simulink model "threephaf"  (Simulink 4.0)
settings: Solver=ode23  StartTime=-eps  StopTime=0.1  FixedStep=0.000001  MaxStep=2e-5  RelTol=1e-3
undefined symbols (not defined in the file or in its folder): Cdc, di, Element, L, R, sfunxy, Symmetrized, Tf, Ts, Udc, Upp, Warning, Yes
libraries: simulink3 x7
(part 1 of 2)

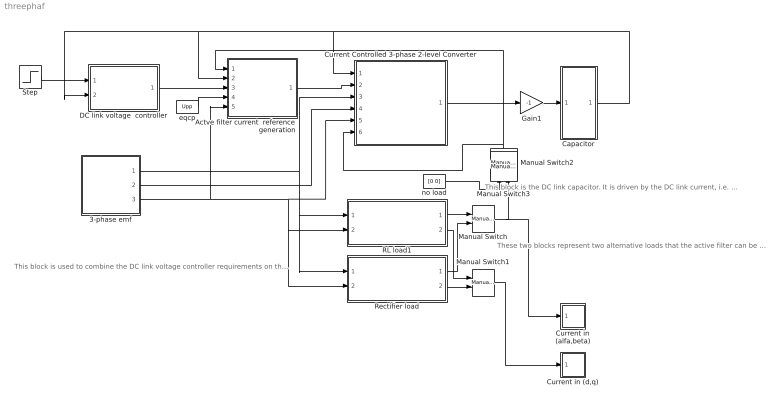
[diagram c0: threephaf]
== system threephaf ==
  note: These two blocks represent two alternative loads that the active filter can be used with.
  note: This block is the DC link capacitor. It is driven by the DC link current, i.e. the DC link voltage is the integral of the DC link current divided by the capacitance.
  note: This block is used to combine the DC link voltage controller requirements on the filter current with the components of the load current that can be filtered out.
  3-phase emf : Subsystem  SimViewingDevice=off  mask{Upp=Upp, freq=50, Tc=0.1e-3}
      mask prompts: Upp "U_phase_to_phase [RMS]"; freq "Frequency"; Tc "Sampling time"
  Actve filter current  reference generation : Subsystem  SimViewingDevice=off
  Capacitor : Subsystem  SimViewingDevice=off
  Current Controlled 3-phase 2-level Converter : Subsystem  SimViewingDevice=off
  Current in (alfa,beta) : Subsystem  LoadFcn=sfunxy([],[],[],'LoadBlock')  StartFcn=sfunxy([],[],[],'Start')  StopFcn=sfunxy([],[],[],'Stop')  SimViewingDevice=off  mask(XY scope.){xmin=-20, xmax=20, ymin=-20, ymax=20, st=-1}
      mask prompts: xmin "x-min:"; xmax "x-max:"; ymin "y-min:"; ymax "y-max:"; st "Sample time:"
      mask help: XY scope using MATLAB graph window. First input is used as time base. Enter plotting ranges.
  Current in (d,q) : Subsystem  LoadFcn=sfunxy([],[],[],'LoadBlock')  StartFcn=sfunxy([],[],[],'Start')  StopFcn=sfunxy([],[],[],'Stop')  SimViewingDevice=off  mask(XY scope.){xmin=-20, xmax=20, ymin=-20, ymax=20, st=-1}
      mask prompts: xmin "x-min:"; xmax "x-max:"; ymin "y-min:"; ymax "y-max:"; st "Sample time:"
      mask help: XY scope using MATLAB graph window. First input is used as time base. Enter plotting ranges.
  DC link voltage  controller : Subsystem  SimViewingDevice=off  mask{Kp=Cdc/3/Tf, Ti=9*Tf, Ttc=Ts, Limitoutput=Yes, Out_max=20, Out_min=-20}
      mask prompts: Kp "Gain"; Ti "Integral time constant"; Ttc "Controller Sampling Time"; Limitoutput "Limit the output"; Out_max "Max Controller Output (if limited)     INCLUDES Anti Windup !!"; Out_min "Min Controller Output (if limited)     INCLUDES Anti Windup !!"
  Gain1 : Gain  Gain=-1  Multiplication=Element-wise(K.*u)  SaturateOnIntegerOverflow=on
  Manual Switch : simulink3/Nonlinear/Manual Switch  sw=0  action=0
  Manual Switch1 : simulink3/Nonlinear/Manual Switch  sw=0  action=0
  Manual Switch2 : simulink3/Nonlinear/Manual Switch  Orientation=up  sw=0  action=0
  Manual Switch3 : simulink3/Nonlinear/Manual Switch  Orientation=up  sw=0  action=0
  RL load1 : Subsystem  SimViewingDevice=off  mask{Ra=5, Rb=5, Rc=5, La=0.005, Lb=0.005, Lc=0.005, Imax=1}
      mask prompts: Ra "Ra [Ohm]"; Rb "Rb [Ohm]"; Rc "Rc [Ohm]"; La "La [H]"; Lb "Lb [H]"; Lc "Lc [H]"; Imax "Current when saturation starts"
  Rectifier load : Subsystem  SimViewingDevice=off
  Step : Step  Time=0.005  Before=250  After=260  SampleTime=0
  eqcp : Constant  Value=Upp
  no load : Constant  Value=[0 0]
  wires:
  Gain1/1 -> Capacitor/1(iC)
  Current Controlled 3-phase 2-level Converter/1(idc) -> Gain1/1
  DC link voltage  controller/1(Out) -> Actve filter current  reference generation/3(idc*)
  eqcp/1 -> Actve filter current  reference generation/4(eqcp)
  Step/1 -> DC link voltage  controller/1(Ref)
  Capacitor/1(Udc) -> Actve filter current  reference generation/2(Udc), DC link voltage  controller/2(Act), Current Controlled 3-phase 2-level Converter/1(Udc)
  RL load1/1(i_load_ab) -> Manual Switch/1
  Rectifier load/1(i_load_ab) -> Manual Switch/2
  Rectifier load/2(i_load_dq) -> Manual Switch1/2
  RL load1/2(i_load_dq) -> Manual Switch1/1
  Actve filter current  reference generation/1(idq*) -> Current Controlled 3-phase 2-level Converter/2(idq*)
  3-phase emf/1(e_line) -> Current Controlled 3-phase 2-level Converter/3(e_line), Rectifier load/1(u_line), RL load1/1(u_line)
  3-phase emf/2(Psi_line) -> Current Controlled 3-phase 2-level Converter/4(Psi_line)
  3-phase emf/3(Theta_line) -> Actve filter current  reference generation/5(Theta), Current Controlled 3-phase 2-level Converter/5(Theta_line), Rectifier load/2(Theta), RL load1/2(Theta)
  Manual Switch/1 -> Manual Switch2/2, Current in (alfa,beta)/1(xy)
  no load/1 -> Manual Switch2/1
  Manual Switch2/1 -> Actve filter current  reference generation/1(i_load), Current Controlled 3-phase 2-level Converter/6(Load current in a/b)
  Manual Switch1/1 -> Current in (d,q)/1(xy)

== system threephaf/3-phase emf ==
  note: Power invariant emf vector on alpha/beta frame
  Cos Fcn : Fcn  Expr=cos(2*pi*(u(2))*u(1))
  Digital Clock : DigitalClock  SampleTime=Tc
  Mux : Mux  Inputs=2
  Mux1 : Mux  Inputs=2
  Product : Product  Inputs=2  Multiplication=Element-wise(.*)  SaturateOnIntegerOverflow=on
  Sine Fcn : Fcn  Expr=sin(2*pi*(u(2))*u(1)-pi)
  frequency : Constant  Value=freq
  integrator : Subsystem  SimViewingDevice=off
  line voltage : Constant  Value=Upp
  rec_to_pol : Subsystem  SimViewingDevice=off
  e_line : Outport  Port=1  InitialOutput=0
  Psi_line : Outport  Port=2  InitialOutput=0
  Theta_line : Outport  Port=3  InitialOutput=0
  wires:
  Product/1 -> e_line/1, integrator/1(In1)
  Mux1/1 -> Product/1
  Cos Fcn/1 -> Mux1/2
  Sine Fcn/1 -> Mux1/1
  Mux/1 -> Cos Fcn/1, Sine Fcn/1
  Digital Clock/1 -> Mux/1
  frequency/1 -> Mux/2
  line voltage/1 -> Product/2
  integrator/1(Out1) -> Psi_line/1, rec_to_pol/1(rect)
  rec_to_pol/2(angle) -> Theta_line/1

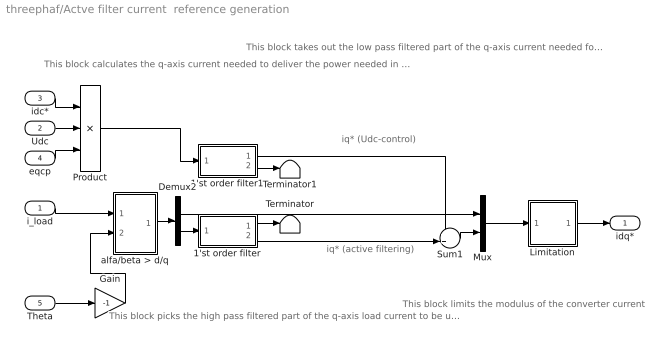
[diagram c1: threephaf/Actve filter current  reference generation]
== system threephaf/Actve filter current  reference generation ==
  note: iq* (Udc-control)
  note: iq* (active filtering)
  note: This block calculates the q-axis current needed to deliver the power needed in the dc-link for correcting the DC link voltage error, as ordered by the DC link voltage controller
  note: This block takes out the low pass filtered part of the q-axis current needed for DC link voltage control
  note: This block picks the high pass filtered part of the q-axis load current to be used as reference for the q-axis together with the low pass filtered part of the DC link voltage controller output.
  note: This block limits the modulus of the converter current
  i_load : Inport  Port=1  PortDimensions=-1  SampleTime=-1  DataType=auto
  Udc : Inport  Port=2  PortDimensions=-1  SampleTime=-1  DataType=auto
  idc* : Inport  Port=3  PortDimensions=-1  SampleTime=-1  DataType=auto
  eqcp : Inport  Port=4  PortDimensions=-1  SampleTime=-1  DataType=auto
  Theta : Inport  Port=5  PortDimensions=-1  SampleTime=-1  DataType=auto
  1'st order filter : Subsystem  SimViewingDevice=off
  1'st order filter1 : Subsystem  SimViewingDevice=off
  Demux2 : Demux  Outputs=2  BusSelectionMode=off
  Gain : Gain  Gain=-1  Multiplication=Element-wise(K.*u)  SaturateOnIntegerOverflow=on
  Limitation : Subsystem  SimViewingDevice=off
  Mux : Mux  Inputs=2
  Product : Product  Inputs=**/  Multiplication=Element-wise(.*)  SaturateOnIntegerOverflow=on
  Sum1 : Sum  Inputs=++|  SaturateOnIntegerOverflow=on
  Terminator : Terminator
  Terminator1 : Terminator
  alfa/beta > d/q : Subsystem  SimViewingDevice=off
  idq* : Outport  Port=1
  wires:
  i_load/1 -> alfa/beta > d/q/1(vect)
  Gain/1 -> alfa/beta > d/q/2(angle)
  Theta/1 -> Gain/1
  Demux2/1 -> Mux/1
  Demux2/2 -> 1'st order filter/1(In)
  1'st order filter/1(OutLP) -> Terminator/1
  alfa/beta > d/q/1(Out) -> Demux2/1
  1'st order filter/2(OutHP) -> Sum1/2
  Sum1/1 -> Mux/2
  Limitation/1(i*lim) -> idq*/1
  1'st order filter1/1(OutLP) -> Sum1/1
  eqcp/1 -> Product/3
  Udc/1 -> Product/2
  Product/1 -> 1'st order filter1/1(In)
  idc*/1 -> Product/1
  1'st order filter1/2(OutHP) -> Terminator1/1
  Mux/1 -> Limitation/1(i*)

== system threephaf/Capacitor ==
  iC : Inport  Port=1  PortDimensions=-1  SampleTime=-1  DataType=auto
  Gain : Gain  Gain=1/Cdc  Multiplication=Element-wise(K.*u)  SaturateOnIntegerOverflow=on
  Integrator : Integrator  ExternalReset=none  InitialConditionSource=internal  InitialCondition=Udc  LimitOutput=off  UpperSaturationLimit=inf  LowerSaturationLimit=-inf  ShowSaturationPort=off  ShowStatePort=off  AbsoluteTolerance=auto
  Udc : Outport  Port=1
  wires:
  Gain/1 -> Integrator/1
  iC/1 -> Gain/1
  Integrator/1 -> Udc/1

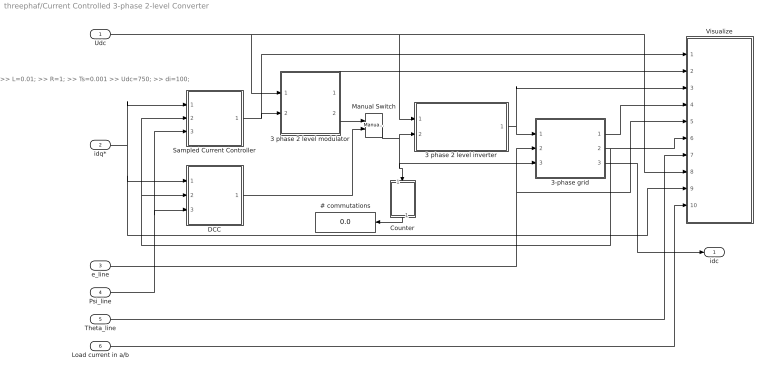
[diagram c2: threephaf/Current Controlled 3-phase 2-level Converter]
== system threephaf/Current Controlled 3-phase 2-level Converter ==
  note: >> L=0.01; >> R=1; >> Ts=0.001 >> Udc=750; >> di=100;
  Udc : Inport  Port=1  PortDimensions=-1  SampleTime=-1  DataType=auto
  idq* : Inport  Port=2  PortDimensions=-1  SampleTime=-1  DataType=auto
  e_line : Inport  Port=3  PortDimensions=-1  SampleTime=-1  DataType=auto
  Psi_line : Inport  Port=4  PortDimensions=-1  SampleTime=-1  DataType=auto
  Theta_line : Inport  Port=5  PortDimensions=-1  SampleTime=-1  DataType=auto
  Load current in a/b : Inport  Port=6  PortDimensions=-1  SampleTime=-1  DataType=auto
  # commutations : Display
  3 phase 2 level inverter : Subsystem  SimViewingDevice=off
  3 phase 2 level modulator : Subsystem  SimViewingDevice=off  mask{type=Symmetrized, Random=Fixed frequency, Ts=Ts}
      mask prompts: type "Sinus, Symmetrized or Minimum switch modulation"; Random "Fixed or random modulation?"; Ts "Sampling interval"
      mask help: Carrier Wave modulator that uses either fixed frequency modulation or random modulation. The fixed frequency modulation uses 1/(2Ts) as modulation frequency. The random modulation selects the modulatio frequency by random every sampling instant. The selection uses either 1/Ts, 1/(2Ts) or 1/(3Ts) as carrier wave frequency.
  3-phase grid : Subsystem  SimViewingDevice=off  mask{L=L, R=R}
      mask prompts: L "Inductance [H]"; R "Resistance [ohm]"
  Counter : Subsystem  Orientation=down  SimViewingDevice=off
  DCC : Subsystem  SimViewingDevice=off
  Manual Switch : simulink3/Nonlinear/Manual Switch  sw=1  action=0
  Sampled Current Controller : Subsystem  SimViewingDevice=off  mask{R=R, L=L, Kp=(L/Ts+R/2), Ti=L/R+Ts/2, Ts=Ts, Umax=Udc, Umin=-Udc, SlowFast=Fast computer}
      mask prompts: R "Load resistance"; L "Load inductance"; Kp "Controller gain"; Ti "Integral Time Constant"; Ts "Sampling time [s]"; Umax "Max output signal"; Umin "Min output signal"; SlowFast "Controller type"
  Visualize : Subsystem  SimViewingDevice=off
  idc : Outport  Port=1
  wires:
  3 phase 2 level inverter/1(va,b,c) -> 3-phase grid/1(va,b,c), Visualize/3(v)
  Sampled Current Controller/1(u*) -> 3 phase 2 level modulator/2(uabc*), Visualize/1(u*)
  Udc/1 -> 3 phase 2 level modulator/1(Udc), 3 phase 2 level inverter/1(Udc), Visualize/8(Udc)
  Counter/1(#) -> # commutations/1
  3 phase 2 level modulator/2(sa,b,c) -> Manual Switch/1
  Manual Switch/1 -> 3 phase 2 level inverter/2(sa,b,c), Counter/1(sa,b,c), 3-phase grid/3(s)
  DCC/1(sa,b,c) -> Manual Switch/2
  3 phase 2 level modulator/1(mod) -> Visualize/2(mod)
  e_line/1 -> 3-phase grid/2(e_line), Visualize/5(e)
  3-phase grid/1(u_ab) -> Visualize/4("u ")
  3-phase grid/2(i_ab) -> Visualize/6(i), DCC/2(Act_ab), Sampled Current Controller/2(Act_ab)
  Theta_line/1 -> Visualize/7(theta)
  Psi_line/1 -> DCC/3(psi), Sampled Current Controller/3(psi)
  idq*/1 -> Sampled Current Controller/1(Ref_dq), DCC/1(Ref_dq), Visualize/9(i*dq)
  3-phase grid/3(i_dc) -> idc/1
  Load current in a/b/1 -> Visualize/10(Load current in a/b)

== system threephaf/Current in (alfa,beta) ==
  xy : Inport  Port=1  PortDimensions=-1  SampleTime=-1  DataType=auto
  sfunxy : S-Function  FunctionName=sfunxy  Parameters=[xmin xmax ymin ymax], st  PortCounts=[]  SFunctionModules=''
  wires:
  xy/1 -> sfunxy/1

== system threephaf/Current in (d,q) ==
  xy : Inport  Port=1  PortDimensions=-1  SampleTime=-1  DataType=auto
  sfunxy : S-Function  FunctionName=sfunxy  Parameters=[xmin xmax ymin ymax], st  PortCounts=[]  SFunctionModules=''
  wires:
  xy/1 -> sfunxy/1

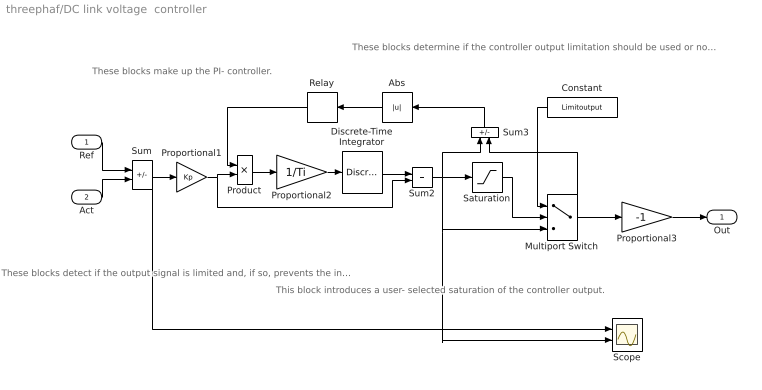
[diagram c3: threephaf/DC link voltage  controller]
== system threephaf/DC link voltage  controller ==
  note: These blocks make up the PI- controller.
  note: These blocks detect if the output signal is limited and, if so, prevents the integrator from integrating.
  note: This block introduces a user- selected saturation of the controller output.
  note: These blocks determine if the controller output limitation should be used or not.
  Ref : Inport  Port=1  PortDimensions=-1  SampleTime=-1  DataType=auto
  Act : Inport  Port=2  PortDimensions=-1  SampleTime=-1  DataType=auto
  Abs : Abs  Orientation=left  SaturateOnIntegerOverflow=on
  Constant : Constant  Orientation=left  Value=Limitoutput
  Discrete-Time Integrator : DiscreteIntegrator  IntegratorMethod=Forward Euler  ExternalReset=none  InitialConditionSource=internal  InitialCondition=0  LimitOutput=off  UpperSaturationLimit=inf  LowerSaturationLimit=-inf  ShowSaturationPort=off  ShowStatePort=off  SampleTime=Ttc
  Multiport Switch : MultiPortSwitch  Inputs=2
  Product : Product  Inputs=2  Multiplication=Element-wise(.*)  SaturateOnIntegerOverflow=on
  Proportional1 : Gain  Gain=Kp  Multiplication=Element-wise(K.*u)  SaturateOnIntegerOverflow=on
  Proportional2 : Gain  Gain=1/Ti  Multiplication=Element-wise(K.*u)  SaturateOnIntegerOverflow=on
  Proportional3 : Gain  Gain=-1  Multiplication=Element-wise(K.*u)  SaturateOnIntegerOverflow=on
  Relay : Relay  Orientation=left  OnSwitchValue=eps  OffSwitchValue=eps  OnOutputValue=0  OffOutputValue=1
  Saturation : Saturate  UpperLimit=Out_max  LowerLimit=Out_min  LinearizeAsGain=on
  Scope : Scope  NumInputPorts=2
  Sum : Sum  Inputs=+-  SaturateOnIntegerOverflow=on
  Sum2 : Sum  Inputs=++  SaturateOnIntegerOverflow=on
  Sum3 : Sum  Orientation=up  Inputs=+-  SaturateOnIntegerOverflow=on
  Out : Outport  Port=1
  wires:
  Sum/1 -> Proportional1/1, Scope/1
  Discrete-Time Integrator/1 -> Sum2/1
  Proportional1/1 -> Product/2, Sum2/2
  Proportional2/1 -> Discrete-Time Integrator/1
  Sum2/1 -> Saturation/1, Sum3/1, Multiport Switch/3, Scope/2
  Product/1 -> Proportional2/1
  Sum3/1 -> Abs/1
  Abs/1 -> Relay/1
  Relay/1 -> Product/1
  Ref/1 -> Sum/1
  Act/1 -> Sum/2
  Saturation/1 -> Multiport Switch/2
  Constant/1 -> Multiport Switch/1
  Multiport Switch/1 -> Sum3/2, Proportional3/1
  Proportional3/1 -> Out/1

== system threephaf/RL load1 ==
  u_line : Inport  Port=1  PortDimensions=-1  SampleTime=-1  DataType=auto
  Theta : Inport  Port=2  PortDimensions=-1  SampleTime=-1  DataType=auto
  Gain1 : Gain  Gain=-1  Multiplication=Element-wise(K.*u)  SaturateOnIntegerOverflow=on
  Load : Subsystem  SimViewingDevice=off  mask{La=La, Lb=Lb, Lc=Lc, Imax=Imax, Ra=Ra, Rb=Rb, Rc=Rc}
      mask prompts: Imax "Inductor current for saturation"
  "a/b -> d/q1" : Subsystem  SimViewingDevice=off
  abc Ü> vector : Subsystem  SimViewingDevice=off
  vector to abc2 : Subsystem  SimViewingDevice=off
  i_load_ab : Outport  Port=1
  i_load_dq : Outport  Port=2
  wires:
  vector to abc2/1(a) -> Load/1(a)
  vector to abc2/2(b) -> Load/2(b)
  vector to abc2/3(c) -> Load/3(c)
  Load/1(ia) -> abc Ü> vector/1(a)
  Load/2(ib) -> abc Ü> vector/2(b)
  Load/3(ic) -> abc Ü> vector/3(c)
  u_line/1 -> vector to abc2/1(vect)
  abc Ü> vector/1(vect) -> i_load_ab/1, "a/b -> d/q1"/1(vect)
  Gain1/1 -> "a/b -> d/q1"/2(angle)
  Theta/1 -> Gain1/1
  "a/b -> d/q1"/1(Out) -> i_load_dq/1

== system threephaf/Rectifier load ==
  u_line : Inport  Port=1  PortDimensions=-1  SampleTime=-1  DataType=auto
  Theta : Inport  Port=2  PortDimensions=-1  SampleTime=-1  DataType=auto
  Gain1 : Gain  Gain=-1  Multiplication=Element-wise(K.*u)  SaturateOnIntegerOverflow=on
  Load : Subsystem  SimViewingDevice=off
  "a/b -> d/q1" : Subsystem  SimViewingDevice=off
  abc Ü> vector : Subsystem  SimViewingDevice=off
  vector to abc2 : Subsystem  SimViewingDevice=off
  i_load_ab : Outport  Port=1
  i_load_dq : Outport  Port=2
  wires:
  "a/b -> d/q1"/1(Out) -> i_load_dq/1
  Theta/1 -> Gain1/1
  Gain1/1 -> "a/b -> d/q1"/2(angle)
  vector to abc2/1(a) -> Load/1(a)
  vector to abc2/2(b) -> Load/2(b)
  vector to abc2/3(c) -> Load/3(c)
  Load/1(ia) -> abc Ü> vector/1(a)
  Load/2(ib) -> abc Ü> vector/2(b)
  Load/3(ic) -> abc Ü> vector/3(c)
  u_line/1 -> vector to abc2/1(vect)
  abc Ü> vector/1(vect) -> "a/b -> d/q1"/1(vect), i_load_ab/1

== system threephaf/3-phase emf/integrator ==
  note: Power invariant emf vector on alpha/beta frame
  In1 : Inport  Port=1  PortDimensions=-1  SampleTime=-1  DataType=auto
  Demux : Demux  Outputs=2  BusSelectionMode=off
  Integrator1 : Integrator  ExternalReset=none  InitialConditionSource=internal  InitialCondition=Upp/(2*pi*freq)  LimitOutput=off  UpperSaturationLimit=inf  LowerSaturationLimit=-inf  ShowSaturationPort=off  ShowStatePort=off  AbsoluteTolerance=auto
  Integrator2 : Integrator  ExternalReset=none  InitialConditionSource=internal  InitialCondition=0  LimitOutput=off  UpperSaturationLimit=inf  LowerSaturationLimit=-inf  ShowSaturationPort=off  ShowStatePort=off  AbsoluteTolerance=auto
  Mux : Mux  Inputs=2
  Out1 : Outport  Port=1
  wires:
  In1/1 -> Demux/1
  Mux/1 -> Out1/1
  Integrator2/1 -> Mux/2
  Integrator1/1 -> Mux/1
  Demux/2 -> Integrator2/1
  Demux/1 -> Integrator1/1

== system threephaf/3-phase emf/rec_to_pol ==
  rect : Inport  Port=1  PortDimensions=-1  SampleTime=-1  DataType=auto
  Derivative : Derivative
  Gain : Gain  Gain=-1  Multiplication=Element-wise(K.*u)  SaturateOnIntegerOverflow=on
  alfa/beta Ü> d/q : Subsystem  SimViewingDevice=off
  "angle " : Fcn  Expr=atan2(u[2],u[1])
  "mod " : Fcn  Expr=sqrt(u[1]^2+u[2]^2)
  e : Outport  Port=1  InitialOutput=0
  angle : Outport  Port=2  InitialOutput=0
  mod : Outport  Port=3  InitialOutput=0
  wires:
  "angle "/1 -> angle/1, Gain/1
  rect/1 -> "angle "/1, "mod "/1, Derivative/1
  "mod "/1 -> mod/1
  Gain/1 -> alfa/beta Ü> d/q/2(angle)
  Derivative/1 -> alfa/beta Ü> d/q/1(vect)
  alfa/beta Ü> d/q/1(Out) -> e/1

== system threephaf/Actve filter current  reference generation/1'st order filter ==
  In : Inport  Port=1  PortDimensions=-1  SampleTime=-1  DataType=auto
  Gain4 : Gain  Gain=1/Tf  Multiplication=Element-wise(K.*u)  SaturateOnIntegerOverflow=on
  Integrator : Integrator  ExternalReset=none  InitialConditionSource=internal  InitialCondition=0  LimitOutput=off  UpperSaturationLimit=inf  LowerSaturationLimit=-inf  ShowSaturationPort=off  ShowStatePort=off  AbsoluteTolerance=auto
  Sum : Sum  Inputs=-+  SaturateOnIntegerOverflow=on
  Sum4 : Sum  Inputs=+-  SaturateOnIntegerOverflow=on
  OutLP : Outport  Port=1
  OutHP : Outport  Port=2
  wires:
  Sum4/1 -> Gain4/1
  Gain4/1 -> Integrator/1
  Integrator/1 -> OutLP/1, Sum4/2, Sum/1
  In/1 -> Sum4/1, Sum/2
  Sum/1 -> OutHP/1

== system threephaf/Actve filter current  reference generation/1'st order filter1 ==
  In : Inport  Port=1  PortDimensions=-1  SampleTime=-1  DataType=auto
  Gain : Gain  Gain=1/(Tf)  Multiplication=Element-wise(K.*u)  SaturateOnIntegerOverflow=on
  Integrator : Integrator  ExternalReset=none  InitialConditionSource=internal  InitialCondition=0  LimitOutput=off  UpperSaturationLimit=inf  LowerSaturationLimit=-inf  ShowSaturationPort=off  ShowStatePort=off  AbsoluteTolerance=auto
  Sum : Sum  Inputs=-+  SaturateOnIntegerOverflow=on
  Sum1 : Sum  Inputs=|+-  SaturateOnIntegerOverflow=on
  OutLP : Outport  Port=1
  OutHP : Outport  Port=2
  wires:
  Sum1/1 -> Gain/1
  Gain/1 -> Integrator/1
  Integrator/1 -> OutLP/1, Sum1/2, Sum/1
  In/1 -> Sum1/1, Sum/2
  Sum/1 -> OutHP/1

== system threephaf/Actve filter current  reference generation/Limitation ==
  note: abs(i*)
  note: Current Limiter
  i* : Inport  Port=1  PortDimensions=-1  SampleTime=-1  DataType=auto
  Constant : Constant  Value=20*sqrt(3/2)
  Fcn1 : Fcn  Expr=sqrt(u(1)^2+u(2)^2)
  Product : Product  Inputs=2  Multiplication=Element-wise(.*)  SaturateOnIntegerOverflow=on
  Product1 : Product  Inputs=2  Multiplication=Element-wise(.*)  SaturateOnIntegerOverflow=on
  Saturation : Saturate  UpperLimit=1  LowerLimit=0  LinearizeAsGain=on
  Sign4 : Signum
  Sum2 : Sum  Inputs=-+  SaturateOnIntegerOverflow=on
  Switch4 : Switch  Threshold=0
  i*lim : Outport  Port=1
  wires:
  Saturation/1 -> Product1/2
  Product/1 -> Saturation/1
  Switch4/1 -> Product/1
  Fcn1/1 -> Product/2, Switch4/3, Sum2/2
  Sum2/1 -> Sign4/1
  Sign4/1 -> Switch4/2
  Constant/1 -> Switch4/1, Sum2/1
  i*/1 -> Product1/1, Fcn1/1
  Product1/1 -> i*lim/1

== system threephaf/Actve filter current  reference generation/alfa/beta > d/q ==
  vect : Inport  Port=1  PortDimensions=-1  SampleTime=-1  DataType=auto
  angle : Inport  Port=2  PortDimensions=-1  SampleTime=-1  DataType=auto
  Fcn : Fcn  Expr=u[1]*cos(u[3])-u[2]*sin(u[3])
  Fcn1 : Fcn  Expr=u[1]*sin(u[3])+u[2]*cos(u[3])
  Mux : Mux  Inputs=2
  Mux1 : Mux  Inputs=2
  Out : Outport  Port=1  InitialOutput=0
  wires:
  vect/1 -> Mux/1
  angle/1 -> Mux/2
  Mux/1 -> Fcn/1, Fcn1/1
  Fcn/1 -> Mux1/1
  Fcn1/1 -> Mux1/2
  Mux1/1 -> Out/1

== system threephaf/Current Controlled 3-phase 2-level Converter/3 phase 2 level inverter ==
  Udc : Inport  Port=1  PortDimensions=-1  SampleTime=-1  DataType=auto
  sa,b,c : Inport  Port=2  PortDimensions=-1  SampleTime=-1  DataType=auto
  Demux : Demux  Outputs=3  BusSelectionMode=off
  Gain : Gain  Gain=1/2  Multiplication=Element-wise(K.*u)  SaturateOnIntegerOverflow=on
  Gain1 : Gain  Gain=-1/2  Multiplication=Element-wise(K.*u)  SaturateOnIntegerOverflow=on
  Mux : Mux  Orientation=down  Inputs=3
  Switch : Switch  Threshold=0
  Switch1 : Switch  Threshold=0
  Switch2 : Switch  Threshold=0
  va,b,c : Outport  Orientation=down  Port=1  InitialOutput=0
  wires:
  Gain/1 -> Switch/1, Switch1/1, Switch2/1
  Gain1/1 -> Switch/3, Switch1/3, Switch2/3
  Udc/1 -> Gain1/1, Gain/1
  sa,b,c/1 -> Demux/1
  Demux/1 -> Switch/2
  Demux/2 -> Switch1/2
  Demux/3 -> Switch2/2
  Switch/1 -> Mux/1
  Switch1/1 -> Mux/2
  Switch2/1 -> Mux/3
  Mux/1 -> va,b,c/1

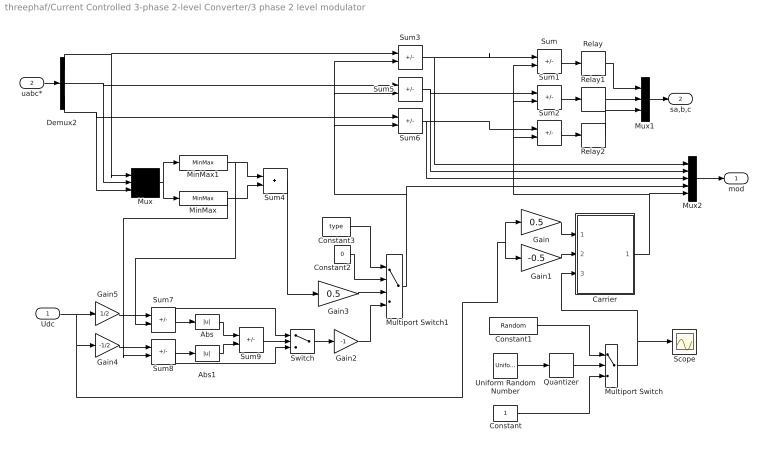
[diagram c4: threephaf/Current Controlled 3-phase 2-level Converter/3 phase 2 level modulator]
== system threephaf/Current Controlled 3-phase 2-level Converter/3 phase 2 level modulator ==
  Udc : Inport  Port=1  PortDimensions=-1  SampleTime=-1  DataType=auto
  uabc* : Inport  Port=2  PortDimensions=-1  SampleTime=-1  DataType=auto
  Abs : Abs  SaturateOnIntegerOverflow=on
  Abs1 : Abs  SaturateOnIntegerOverflow=on
  Carrier : Subsystem  SimViewingDevice=off
  Constant : Constant  Value=1
  Constant1 : Constant  Value=Random
  Constant2 : Constant  Value=0
  Constant3 : Constant  Value=type
  Demux2 : Demux  Outputs=3  BusSelectionMode=off
  Gain : Gain  Gain=0.5  Multiplication=Element-wise(K.*u)  SaturateOnIntegerOverflow=on
  Gain1 : Gain  Gain=-0.5  Multiplication=Element-wise(K.*u)  SaturateOnIntegerOverflow=on
  Gain2 : Gain  Gain=-1  Multiplication=Element-wise(K.*u)  SaturateOnIntegerOverflow=on
  Gain3 : Gain  Gain=0.5  Multiplication=Element-wise(K.*u)  SaturateOnIntegerOverflow=on
  Gain4 : Gain  Gain=-1/2  Multiplication=Element-wise(K.*u)  SaturateOnIntegerOverflow=on
  Gain5 : Gain  Gain=1/2  Multiplication=Element-wise(K.*u)  SaturateOnIntegerOverflow=on
  MinMax : MinMax  Function=min  Inputs=1
  MinMax1 : MinMax  Function=max  Inputs=1
  Multiport Switch : MultiPortSwitch  Inputs=2
  Multiport Switch1 : MultiPortSwitch  Inputs=3
  Mux : Mux  Inputs=3
  Mux1 : Mux  Inputs=3
  Mux2 : Mux  Inputs=5
  Quantizer : Quantizer  QuantizationInterval=1  LinearizeAsGain=on
  Relay : Relay  OnSwitchValue=eps  OffSwitchValue=eps  OnOutputValue=1  OffOutputValue=-1
  Relay1 : Relay  OnSwitchValue=eps  OffSwitchValue=eps  OnOutputValue=1  OffOutputValue=-1
  Relay2 : Relay  OnSwitchValue=eps  OffSwitchValue=eps  OnOutputValue=1  OffOutputValue=-1
  Scope : Scope
  Sum{,1..3,5..8} (8 alike) : Sum  Inputs=+-  SaturateOnIntegerOverflow=on
  Sum4 : Sum  Inputs=++  SaturateOnIntegerOverflow=on
  Sum9 : Sum  Inputs=-+  SaturateOnIntegerOverflow=on
  Switch : Switch  Threshold=0
  Uniform Random Number : UniformRandomNumber  Minimum=1  Maximum=3  Seed=0.9874  SampleTime=Ts
  mod : Outport  Port=1  InitialOutput=0
  sa,b,c : Outport  Port=2  InitialOutput=0
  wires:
  Carrier/1(um) -> Sum2/2, Sum1/2, Sum/2, Mux2/5
  Gain1/1 -> Carrier/2(Umin)
  Gain/1 -> Carrier/1(Umax)
  Sum/1 -> Relay/1
  Relay1/1 -> Mux1/2
  Sum1/1 -> Relay1/1
  Relay2/1 -> Mux1/3
  Sum2/1 -> Relay2/1
  Quantizer/1 -> Multiport Switch/2
  Uniform Random Number/1 -> Quantizer/1
  Constant/1 -> Multiport Switch/3
  Multiport Switch/1 -> Carrier/3(x), Scope/1
  Constant1/1 -> Multiport Switch/1
  Sum3/1 -> Mux2/1, Sum/1
  Sum5/1 -> Mux2/2, Sum1/1
  Sum6/1 -> Mux2/3, Sum2/1
  Demux2/1 -> Sum3/1, Mux/1
  Demux2/2 -> Sum5/1, Mux/2
  Demux2/3 -> Sum6/1, Mux/3
  Mux/1 -> MinMax1/1, MinMax/1
  MinMax1/1 -> Sum4/1, Sum7/2
  MinMax/1 -> Sum4/2, Sum8/2
  Udc/1 -> Gain5/1, Gain4/1, Gain1/1, Gain/1
  Gain4/1 -> Sum8/1
  Sum7/1 -> Abs/1, Switch/1
  Sum8/1 -> Abs1/1, Switch/3
  Abs/1 -> Sum9/1
  Abs1/1 -> Sum9/2
  Sum9/1 -> Switch/2
  Sum4/1 -> Gain3/1
  Switch/1 -> Gain2/1
  Constant3/1 -> Multiport Switch1/1
  Constant2/1 -> Multiport Switch1/2
  Gain3/1 -> Multiport Switch1/3
  Gain2/1 -> Multiport Switch1/4
  Multiport Switch1/1 -> Sum5/2, Sum3/2, Sum6/2, Mux2/4
  Gain5/1 -> Sum7/1
  uabc*/1 -> Demux2/1
  Relay/1 -> Mux1/1
  Mux1/1 -> sa,b,c/1
  Mux2/1 -> mod/1

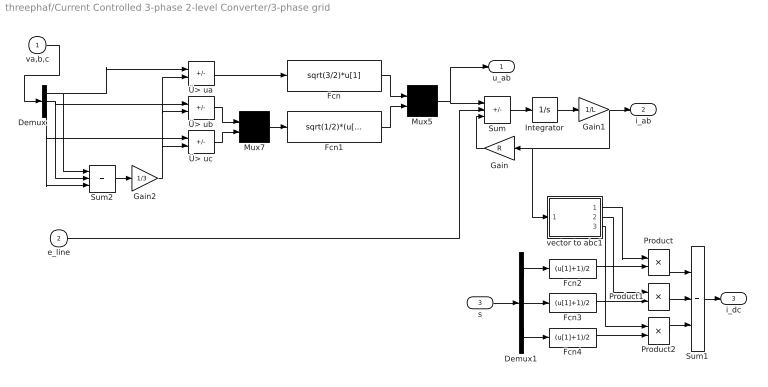
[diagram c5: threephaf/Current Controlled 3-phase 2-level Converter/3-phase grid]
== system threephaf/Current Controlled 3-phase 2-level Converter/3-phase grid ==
  va,b,c : Inport  Port=1  PortDimensions=-1  SampleTime=-1  DataType=auto
  e_line : Inport  Port=2  PortDimensions=-1  SampleTime=-1  DataType=auto
  s : Inport  Port=3  PortDimensions=-1  SampleTime=-1  DataType=auto
  Demux : Demux  Outputs=3  BusSelectionMode=off
  Demux1 : Demux  Outputs=3  BusSelectionMode=off
  Fcn : Fcn  Expr=sqrt(3/2)*u[1]
  Fcn1 : Fcn  Expr=sqrt(1/2)*(u[1]-u[2])
  Fcn2 : Fcn  Expr=(u[1]+1)/2
  Fcn3 : Fcn  Expr=(u[1]+1)/2
  Fcn4 : Fcn  Expr=(u[1]+1)/2
  Gain : Gain  Orientation=left  Gain=R  Multiplication=Element-wise(K.*u)  SaturateOnIntegerOverflow=on
  Gain1 : Gain  Gain=1/L  Multiplication=Element-wise(K.*u)  SaturateOnIntegerOverflow=on
  Gain2 : Gain  Gain=1/3  Multiplication=Element-wise(K.*u)  SaturateOnIntegerOverflow=on
  Integrator : Integrator  ExternalReset=none  InitialConditionSource=internal  InitialCondition=0  LimitOutput=off  UpperSaturationLimit=inf  LowerSaturationLimit=-inf  ShowSaturationPort=off  ShowStatePort=off  AbsoluteTolerance=auto
  Mux5 : Mux  Inputs=2
  Mux7 : Mux  Inputs=2
  Product : Product  Inputs=2  Multiplication=Element-wise(.*)  SaturateOnIntegerOverflow=on
  Product1 : Product  Inputs=2  Multiplication=Element-wise(.*)  SaturateOnIntegerOverflow=on
  Product2 : Product  Inputs=2  Multiplication=Element-wise(.*)  SaturateOnIntegerOverflow=on
  Sum : Sum  Inputs=+--  SaturateOnIntegerOverflow=on
  Sum1 : Sum  Inputs=+++  SaturateOnIntegerOverflow=on
  Sum2 : Sum  Inputs=+++  SaturateOnIntegerOverflow=on
  vector to abc1 : Subsystem  SimViewingDevice=off
  Ü> ua : Sum  Inputs=+-  SaturateOnIntegerOverflow=on
  Ü> ub : Sum  Inputs=+-  SaturateOnIntegerOverflow=on
  Ü> uc : Sum  Inputs=+-  SaturateOnIntegerOverflow=on
  u_ab : Outport  Port=1  InitialOutput=0
  i_ab : Outport  Port=2  InitialOutput=0
  i_dc : Outport  Port=3
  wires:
  Gain1/1 -> i_ab/1, Gain/1, vector to abc1/1(vect)
  Integrator/1 -> Gain1/1
  Gain/1 -> Sum/3
  Sum/1 -> Integrator/1
  Fcn1/1 -> Mux5/2
  Fcn/1 -> Mux5/1
  Mux5/1 -> Sum/1, u_ab/1
  Mux7/1 -> Fcn1/1
  Ü> uc/1 -> Mux7/2
  Ü> ub/1 -> Mux7/1
  Ü> ua/1 -> Fcn/1
  Gain2/1 -> Ü> uc/2, Ü> ub/2, Ü> ua/2
  Demux/2 -> Ü> ub/1, Sum2/2
  Sum2/1 -> Gain2/1
  Demux/3 -> Ü> uc/1, Sum2/3
  Demux/1 -> Ü> ua/1, Sum2/1
  va,b,c/1 -> Demux/1
  Demux1/2 -> Fcn3/1
  Demux1/1 -> Fcn2/1
  Demux1/3 -> Fcn4/1
  s/1 -> Demux1/1
  Sum1/1 -> i_dc/1
  Product2/1 -> Sum1/3
  Product1/1 -> Sum1/2
  Product/1 -> Sum1/1
  vector to abc1/1(a) -> Product/1
  vector to abc1/2(b) -> Product1/1
  vector to abc1/3(c) -> Product2/1
  Fcn4/1 -> Product2/2
  Fcn3/1 -> Product1/2
  Fcn2/1 -> Product/2
  e_line/1 -> Sum/2

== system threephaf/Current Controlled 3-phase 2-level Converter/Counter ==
  sa,b,c : Inport  Port=1  PortDimensions=-1  SampleTime=-1  DataType=auto
  Demux : Demux  Outputs=3  BusSelectionMode=off
  Subsystem : Subsystem  TreatAsAtomicUnit=on  SimViewingDevice=off
  Subsystem1 : Subsystem  TreatAsAtomicUnit=on  SimViewingDevice=off
  Subsystem2 : Subsystem  TreatAsAtomicUnit=on  SimViewingDevice=off
  Sum : Sum  Inputs=+++  SaturateOnIntegerOverflow=on
  # : Outport  Port=1
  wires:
  Sum/1 -> #/1
  Subsystem/1(Out1) -> Sum/2
  Subsystem2/1(Out1) -> Sum/1
  Subsystem1/1(Out1) -> Sum/3
  sa,b,c/1 -> Demux/1
  Demux/2 -> Subsystem/Trigger
  Demux/3 -> Subsystem1/Trigger
  Demux/1 -> Subsystem2/Trigger

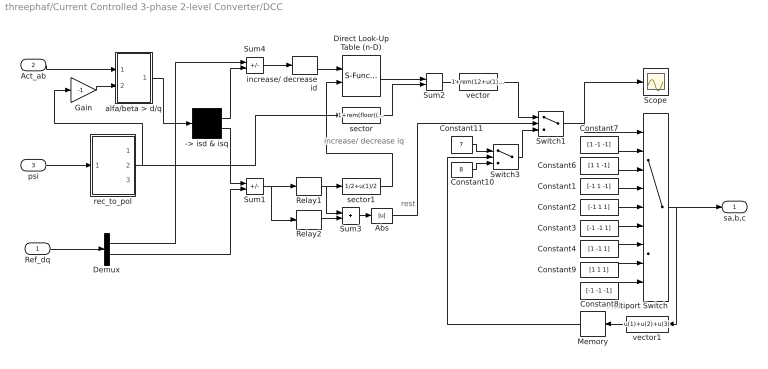
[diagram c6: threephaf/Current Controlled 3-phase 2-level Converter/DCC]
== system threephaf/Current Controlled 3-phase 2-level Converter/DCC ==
  note: increase/ decrease iq
  note: rest
  Ref_dq : Inport  Port=1  PortDimensions=-1  SampleTime=-1  DataType=auto
  Act_ab : Inport  Port=2  PortDimensions=-1  SampleTime=-1  DataType=auto
  psi : Inport  Port=3  PortDimensions=-1  SampleTime=-1  DataType=auto
  -> isd & isq : Demux  Outputs=2  BusSelectionMode=off
  Abs : Abs  SaturateOnIntegerOverflow=on
  Constant1 : Constant  Value=[-1 1 -1]
  Constant10 : Constant  Value=8
  Constant11 : Constant  Value=7
  Constant2 : Constant  Value=[-1 1 1]
  Constant3 : Constant  Value=[-1 -1 1]
  Constant4 : Constant  Value=[1 -1 1]
  Constant6 : Constant  Value=[1 1 -1]
  Constant7 : Constant  Value=[1 -1 -1]
  Constant8 : Constant  Value=[-1 -1 -1]
  Constant9 : Constant  Value=[1 1 1]
  Demux : Demux  Outputs=2  BusSelectionMode=off
  Direct Look-Up Table (n-D) : S-Function  FunctionName=sfun_nddirectlook  Parameters=numInputs,mxTable,clipFlag,tabIsInput,numTDims  PortCounts=[]  SFunctionModules=''  mask(LookupNDDirect){maskTabDims=2, explicitNumDims=1, outDims=Element, tabIsInput=off, mxTable=[4 2;5 1], clipFlag=Warning}
      mask prompts: maskTabDims "Number of table dimensions:"; explicitNumDims "Explicit number of table dimensions:"; outDims "Inputs select this object from table:"; tabIsInput "Make table an input"; mxTable "Table data:"; clipFlag "Action for out of range input:"
      mask help: Table member selection. Inputs are zero-based indices into the table, e.g., an input of 3 returns the fourth element in that dimension. Block can also be used to select a column or 2-D matrix out of the table.
      mask init:
      | if tabIsInput == 1
      |   tWhat = ' T';
      |   yT = 1/(3+maskTabDims-outDims);
      | else
      |   tWhat = ' ';
      |   yT = 0;
      | end
      | if maskTabDims >= 5
      |   numTDims = explicitNumDims;
      | else
      |   numTDims = maskTabDims;
      | end
      | numInputs =  numTDims - (outDims-1);
      | if strcmp(get_param(bdroot(gcb),'BlockDiagramType'),'library')
      |   dimsChar = 'n';
      | else
      |   dimsChar = sprintf('%d',numTDims);
      | end
      | [x,y] = nddirectico('plotdata', numTDims, tabIsInput, outDims);
      | xp = x((end-3):end); yp = y((end-3):end);
      | x = x(1:(end-4)); y = y(1:(end-4));
  Gain : Gain  Gain=-1  Multiplication=Element-wise(K.*u)  SaturateOnIntegerOverflow=on
  Memory : Memory  Orientation=left  X0=0  InheritSampleTime=off
  Multiport Switch : MultiPortSwitch  Inputs=8
  Relay1 : Relay  OnSwitchValue=di/2  OffSwitchValue=-di/2  OnOutputValue=1  OffOutputValue=-1
  Relay2 : Relay  OnSwitchValue=1.3*di/2  OffSwitchValue=-1.3*di/2  OnOutputValue=1  OffOutputValue=-1
  Scope : Scope
  Sum1 : Sum  Inputs=-+  SaturateOnIntegerOverflow=on
  Sum2 : Sum  Inputs=++  SaturateOnIntegerOverflow=on
  Sum3 : Sum  Inputs=++  SaturateOnIntegerOverflow=on
  Sum4 : Sum  Inputs=+-  SaturateOnIntegerOverflow=on
  Switch1 : Switch  Threshold=1
  Switch3 : Switch  Threshold=1
  alfa/beta > d/q : Subsystem  SimViewingDevice=off
  increase/ decrease id : Relay  OnSwitchValue=di/2  OffSwitchValue=-di/2  OnOutputValue=1  OffOutputValue=0
  rec_to_pol : Subsystem  SimViewingDevice=off
  sector : Fcn  Expr=1+rem(floor((2*pi+u(1)+pi/6)/(pi/3+eps)),6)
  sector1 : Fcn  Expr=1/2+u(1)/2
  vector : Fcn  Expr=1+rem(12+u(1)-1,6)
  vector1 : Fcn  Orientation=left  Expr=u(1)+u(2)+u(3)
  sa,b,c : Outport  Port=1
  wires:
  Gain/1 -> alfa/beta > d/q/2(angle)
  Act_ab/1 -> alfa/beta > d/q/1(vect)
  alfa/beta > d/q/1(Out) -> -> isd & isq/1
  psi/1 -> rec_to_pol/1(rect)
  -> isd & isq/1 -> Sum4/2
  rec_to_pol/2(angle) -> Gain/1, sector/1
  Multiport Switch/1 -> vector1/1, sa,b,c/1
  Switch1/1 -> Multiport Switch/1, Scope/1
  vector/1 -> Switch1/1
  Sum4/1 -> increase/ decrease id/1
  Sum2/1 -> vector/1
  vector1/1 -> Memory/1
  -> isd & isq/2 -> Sum1/1
  Constant10/1 -> Switch3/3
  Constant11/1 -> Switch3/1
  Memory/1 -> Switch3/2
  Switch3/1 -> Switch1/3
  Relay1/1 -> Sum3/1, sector1/1
  Relay2/1 -> Sum3/2
  Sum3/1 -> Abs/1
  Sum1/1 -> Relay1/1, Relay2/1
  Abs/1 -> Switch1/2
  increase/ decrease id/1 -> Direct Look-Up Table (n-D)/1
  sector1/1 -> Direct Look-Up Table (n-D)/2
  sector/1 -> Sum2/2
  Direct Look-Up Table (n-D)/1 -> Sum2/1
  Constant6/1 -> Multiport Switch/3
  Constant7/1 -> Multiport Switch/2
  Constant8/1 -> Multiport Switch/9
  Constant9/1 -> Multiport Switch/8
  Constant1/1 -> Multiport Switch/4
  Constant2/1 -> Multiport Switch/5
  Constant3/1 -> Multiport Switch/6
  Constant4/1 -> Multiport Switch/7
  Ref_dq/1 -> Demux/1
  Demux/1 -> Sum4/1
  Demux/2 -> Sum1/2

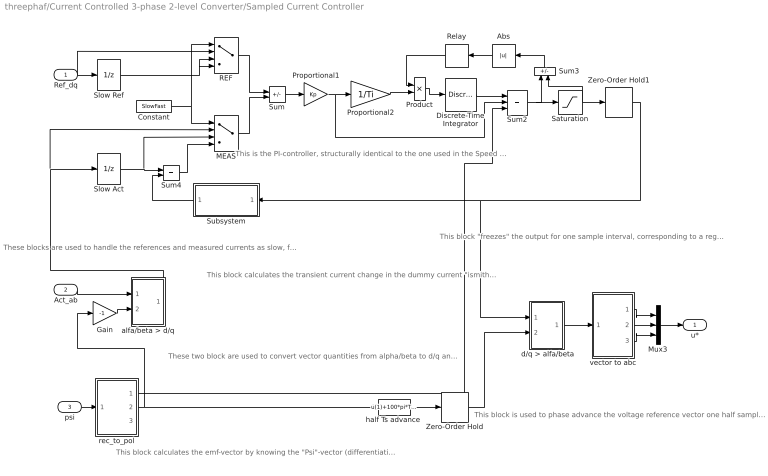
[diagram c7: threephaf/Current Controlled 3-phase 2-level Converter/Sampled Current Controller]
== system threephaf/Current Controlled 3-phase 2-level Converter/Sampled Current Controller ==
  note: These blocks are used to handle the references and measured currents as slow, fast or fast computer with Smith predictor.
  note: This block calculates the transient current change in the dummy current "ismith" The smith predictor calculates the current change that would have been measured if the computer was "fast", i.e. without the delay that a slow computer has. The calculated current change equals the real current change, but informing the controller one sampling interval earlier, thus allowing a high (deadbeat) gain.
  note: This is the PI-controller, structurally identical to the one used in the Speed Controller
  note: This block "freezes" the output for one sample interval, corresponding to a register in a microcontroller where the reference voltages are written once every sampling inteval.
  note: These two block are used to convert vector quantities from alpha/beta to d/q and back again. Note that they are identical, but use the angle with opposite sign.
  note: This block calculates the emf-vector by knowing the "Psi"-vector (differentiation) and calculates the emf- components in the d/q-plane (ideally there is only "eq" whilse "ed"=0). It alse calculates the angle of the "Psi"- vector, used to orient the d/q-plane.
  note: This block is used to phase advance the voltage reference vector one half sample period. It is done to compensate for the fact that the "reality" is turning during the same sample period as the voltage references are being held constant. In the beginning of the sample period, the voltage reference will be 1/2 sample period ahead of reality, and in the end of the sample period it will be 1/2 period behind. In average, it will be in the correct position relative to reality.
  Ref_dq : Inport  Port=1  PortDimensions=-1  SampleTime=-1  DataType=auto
  Act_ab : Inport  Port=2  PortDimensions=-1  SampleTime=-1  DataType=auto
  psi : Inport  Port=3  PortDimensions=-1  SampleTime=-1  DataType=auto
  " d/q > alfa/beta" : Subsystem  SimViewingDevice=off
  Abs : Abs  Orientation=left  SaturateOnIntegerOverflow=on
  Constant : Constant  Value=SlowFast
  Discrete-Time Integrator : DiscreteIntegrator  IntegratorMethod=Forward Euler  ExternalReset=none  InitialConditionSource=internal  InitialCondition=0  LimitOutput=on  UpperSaturationLimit=Umax  LowerSaturationLimit=Umin  ShowSaturationPort=off  ShowStatePort=off  SampleTime=Ts
  Gain : Gain  Gain=-1  Multiplication=Element-wise(K.*u)  SaturateOnIntegerOverflow=on
  MEAS : MultiPortSwitch  Inputs=3
  Mux3 : Mux  Inputs=3
  Product : Product  Inputs=2  Multiplication=Element-wise(.*)  SaturateOnIntegerOverflow=on
  Proportional1 : Gain  Gain=Kp  Multiplication=Element-wise(K.*u)  SaturateOnIntegerOverflow=on
  Proportional2 : Gain  Gain=1/Ti  Multiplication=Element-wise(K.*u)  SaturateOnIntegerOverflow=on
  REF : MultiPortSwitch  Inputs=3
  Relay : Relay  Orientation=left  OnSwitchValue=eps  OffSwitchValue=eps  OnOutputValue=0  OffOutputValue=1
  Saturation : Saturate  UpperLimit=Umax  LowerLimit=Umin  LinearizeAsGain=on
  Slow Act : UnitDelay  X0=0  SampleTime=Ts
  Slow Ref : UnitDelay  X0=0  SampleTime=Ts
  Subsystem : Subsystem  Orientation=left  SimViewingDevice=off
  Sum : Sum  Inputs=+-  SaturateOnIntegerOverflow=on
  Sum2 : Sum  Inputs=+++  SaturateOnIntegerOverflow=on
  Sum3 : Sum  Orientation=up  Inputs=+-  SaturateOnIntegerOverflow=on
  Sum4 : Sum  Inputs=++  SaturateOnIntegerOverflow=on
  Zero-Order Hold : ZeroOrderHold  SampleTime=Ts
  Zero-Order Hold1 : ZeroOrderHold  SampleTime=Ts
  alfa/beta > d/q : Subsystem  SimViewingDevice=off
  "half Ts advance " : Fcn  Expr=u(1)+100*pi*Ts/2
  rec_to_pol : Subsystem  SimViewingDevice=off
  vector to abc : Subsystem  SimViewingDevice=off
  u* : Outport  Port=1
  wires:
  Discrete-Time Integrator/1 -> Sum2/1
  Proportional1/1 -> Proportional2/1, Sum2/2
  Sum/1 -> Proportional1/1
  Sum2/1 -> Saturation/1, Sum3/1
  Saturation/1 -> Zero-Order Hold1/1, Sum3/2
  Proportional2/1 -> Product/2
  Product/1 -> Discrete-Time Integrator/1
  Relay/1 -> Product/1
  Ref_dq/1 -> REF/2, Slow Ref/1
  Zero-Order Hold1/1 -> Subsystem/1(u), " d/q > alfa/beta"/1(vect)
  Slow Act/1 -> Sum4/1, MEAS/3
  Subsystem/1(di_smith) -> Sum4/2
  Constant/1 -> MEAS/1, REF/1
  Slow Ref/1 -> REF/3, REF/4
  REF/1 -> Sum/1
  Sum4/1 -> MEAS/4
  MEAS/1 -> Sum/2
  Sum3/1 -> Abs/1
  Abs/1 -> Relay/1
  Gain/1 -> alfa/beta > d/q/2(angle)
  Act_ab/1 -> alfa/beta > d/q/1(vect)
  psi/1 -> rec_to_pol/1(rect)
  rec_to_pol/2(angle) -> Gain/1, "half Ts advance "/1
  "half Ts advance "/1 -> Zero-Order Hold/1
  Zero-Order Hold/1 -> " d/q > alfa/beta"/2(angle)
  " d/q > alfa/beta"/1(Out) -> vector to abc/1(vect)
  vector to abc/1(a) -> Mux3/1
  vector to abc/2(b) -> Mux3/2
  vector to abc/3(c) -> Mux3/3
  alfa/beta > d/q/1(Out) -> Slow Act/1, MEAS/2
  Mux3/1 -> u*/1
  rec_to_pol/1(e) -> Sum2/3

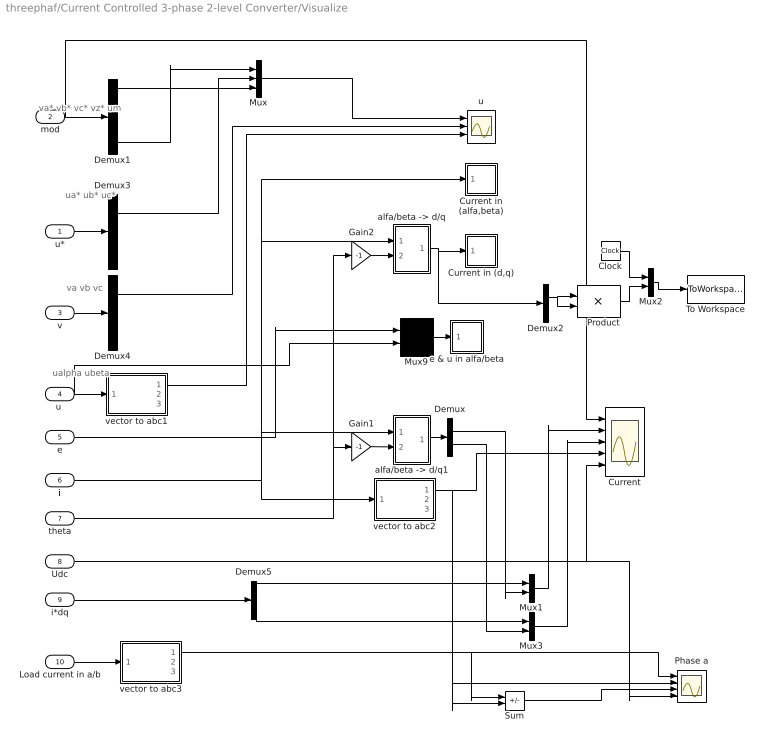
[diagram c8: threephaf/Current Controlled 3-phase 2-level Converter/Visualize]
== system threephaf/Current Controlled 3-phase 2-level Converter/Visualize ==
  note: va* vb* vc* vz* um
  note: ua* ub* uc*
  note: ualpha ubeta
  note: va vb vc
  u* : Inport  Port=1  PortDimensions=-1  SampleTime=-1  DataType=auto
  mod : Inport  Port=2  PortDimensions=-1  SampleTime=-1  DataType=auto
  v : Inport  Port=3  PortDimensions=-1  SampleTime=-1  DataType=auto
  "u " : Inport  Port=4  PortDimensions=-1  SampleTime=-1  DataType=auto
  e : Inport  Port=5  PortDimensions=-1  SampleTime=-1  DataType=auto
  i : Inport  Port=6  PortDimensions=-1  SampleTime=-1  DataType=auto
  theta : Inport  Port=7  PortDimensions=-1  SampleTime=-1  DataType=auto
  Udc : Inport  Port=8  PortDimensions=-1  SampleTime=-1  DataType=auto
  i*dq : Inport  Port=9  PortDimensions=-1  SampleTime=-1  DataType=auto
  Load current in a/b : Inport  Port=10  PortDimensions=-1  SampleTime=-1  DataType=auto
  Clock : Clock
  Current : Scope  NumInputPorts=5
  Current in (alfa,beta) : Subsystem  LoadFcn=sfunxy([],[],[],'LoadBlock')  StartFcn=sfunxy([],[],[],'Start')  StopFcn=sfunxy([],[],[],'Stop')  SimViewingDevice=off  mask(XY scope.){xmin=-20, xmax=20, ymin=-20, ymax=20, st=-1}
      mask prompts: xmin "x-min:"; xmax "x-max:"; ymin "y-min:"; ymax "y-max:"; st "Sample time:"
      mask help: XY scope using MATLAB graph window. First input is used as time base. Enter plotting ranges.
  Current in (d,q) : Subsystem  LoadFcn=sfunxy([],[],[],'LoadBlock')  StartFcn=sfunxy([],[],[],'Start')  StopFcn=sfunxy([],[],[],'Stop')  SimViewingDevice=off  mask(XY scope.){xmin=-20, xmax=20, ymin=-20, ymax=20, st=-1}
      mask prompts: xmin "x-min:"; xmax "x-max:"; ymin "y-min:"; ymax "y-max:"; st "Sample time:"
      mask help: XY scope using MATLAB graph window. First input is used as time base. Enter plotting ranges.
  Demux : Demux  Outputs=2  BusSelectionMode=off
  Demux1 : Demux  Outputs=5  BusSelectionMode=off
  Demux2 : Demux  Outputs=2  BusSelectionMode=off
  Demux3 : Demux  Outputs=3  BusSelectionMode=off
  Demux4 : Demux  Outputs=3  BusSelectionMode=off
  Demux5 : Demux  Outputs=2  BusSelectionMode=off
  Gain1 : Gain  Gain=-1  Multiplication=Element-wise(K.*u)  SaturateOnIntegerOverflow=on
  Gain2 : Gain  Gain=-1  Multiplication=Element-wise(K.*u)  SaturateOnIntegerOverflow=on
  Mux : Mux  Inputs=3
  Mux{1..3,9} (4 alike) : Mux  Inputs=2
  Phase a : Scope  NumInputPorts=4
  Product : Product  Inputs=2  Multiplication=Element-wise(.*)  SaturateOnIntegerOverflow=on
  Sum : Sum  Inputs=+-  SaturateOnIntegerOverflow=on
  To Workspace : ToWorkspace  VariableName=f1  SampleTime=-1  SaveFormat=Array
  "alfa/beta -> d/q" : Subsystem  SimViewingDevice=off
  "alfa/beta -> d/q1" : Subsystem  SimViewingDevice=off
  e & u in alfa/beta : Subsystem  LoadFcn=sfunxy([],[],[],'LoadBlock')  StartFcn=sfunxy([],[],[],'Start')  StopFcn=sfunxy([],[],[],'Stop')  SimViewingDevice=off  mask(XY scope.){xmin=-300, xmax=300, ymin=-300, ymax=300, st=-1}
      mask prompts: xmin "x-min:"; xmax "x-max:"; ymin "y-min:"; ymax "y-max:"; st "Sample time:"
      mask help: XY scope using MATLAB graph window. First input is used as time base. Enter plotting ranges.
  u : Scope  NumInputPorts=3
  vector to abc1 : Subsystem  SimViewingDevice=off
  vector to abc2 : Subsystem  SimViewingDevice=off
  vector to abc3 : Subsystem  SimViewingDevice=off
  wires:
  Gain2/1 -> "alfa/beta -> d/q"/2(angle)
  Gain1/1 -> "alfa/beta -> d/q1"/2(angle)
  "alfa/beta -> d/q1"/1(Out) -> Demux/1
  vector to abc2/1(a) -> Current/4, Phase a/2, Sum/2
  mod/1 -> Demux1/1, Current/1
  "alfa/beta -> d/q"/1(Out) -> Current in (d,q)/1(xy), Demux2/1
  Demux1/5 -> Mux/1
  Demux1/1 -> Mux/3
  Mux/1 -> u/1
  u*/1 -> Demux3/1
  "u "/1 -> vector to abc1/1(vect), Mux9/2
  Demux3/1 -> Mux/2
  v/1 -> Demux4/1
  Demux4/1 -> u/2
  vector to abc1/1(a) -> u/3
  i/1 -> Current in (alfa,beta)/1(xy), "alfa/beta -> d/q"/1(vect), "alfa/beta -> d/q1"/1(vect), vector to abc2/1(vect)
  Mux9/1 -> e & u in alfa/beta/1(xy)
  e/1 -> Mux9/1
  theta/1 -> Gain1/1, Gain2/1
  Clock/1 -> Mux2/1
  Product/1 -> Mux2/2
  Mux2/1 -> To Workspace/1
  Demux2/1 -> Product/1, Product/2
  Udc/1 -> Current/5, Phase a/4
  i*dq/1 -> Demux5/1
  Demux5/1 -> Mux1/1
  Demux5/2 -> Mux3/1
  Demux/1 -> Mux1/2
  Demux/2 -> Mux3/2
  Mux1/1 -> Current/2
  Mux3/1 -> Current/3
  Load current in a/b/1 -> vector to abc3/1(vect)
  vector to abc3/1(a) -> Phase a/1, Sum/1
  Sum/1 -> Phase a/3

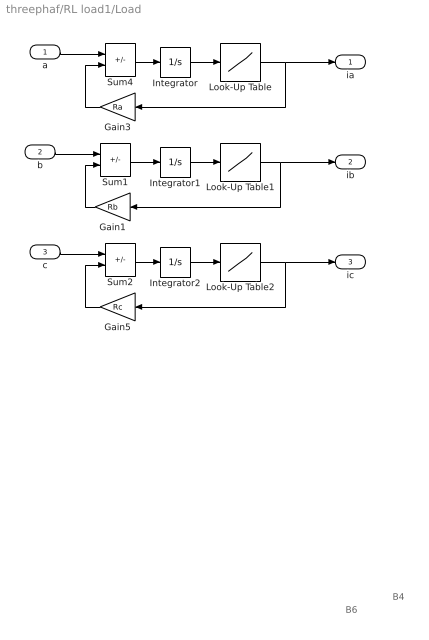
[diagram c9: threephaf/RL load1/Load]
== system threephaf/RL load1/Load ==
  note: B4
  note: B6
  a : Inport  Port=1  PortDimensions=-1  SampleTime=-1  DataType=auto
  b : Inport  Port=2  PortDimensions=-1  SampleTime=-1  DataType=auto
  c : Inport  Port=3  PortDimensions=-1  SampleTime=-1  DataType=auto
  Gain1 : Gain  Orientation=left  Gain=Rb  Multiplication=Element-wise(K.*u)  SaturateOnIntegerOverflow=on
  Gain3 : Gain  Orientation=left  Gain=Ra  Multiplication=Element-wise(K.*u)  SaturateOnIntegerOverflow=on
  Gain5 : Gain  Orientation=left  Gain=Rc  Multiplication=Element-wise(K.*u)  SaturateOnIntegerOverflow=on
  Integrator : Integrator  ExternalReset=none  InitialConditionSource=internal  InitialCondition=0  LimitOutput=off  UpperSaturationLimit=inf  LowerSaturationLimit=-inf  ShowSaturationPort=off  ShowStatePort=off  AbsoluteTolerance=auto
  Integrator1 : Integrator  ExternalReset=none  InitialConditionSource=internal  InitialCondition=0  LimitOutput=off  UpperSaturationLimit=inf  LowerSaturationLimit=-inf  ShowSaturationPort=off  ShowStatePort=off  AbsoluteTolerance=auto
  Integrator2 : Integrator  ExternalReset=none  InitialConditionSource=internal  InitialCondition=0  LimitOutput=off  UpperSaturationLimit=inf  LowerSaturationLimit=-inf  ShowSaturationPort=off  ShowStatePort=off  AbsoluteTolerance=auto
  Look-Up Table : Lookup  InputValues=La*Imax*[-2 -1.5 -1 0 1 1.5 2]  OutputValues=Imax*[-10 -2 -1 0 1 2 10]
  Look-Up Table1 : Lookup  InputValues=Lb*Imax*[-2 -1.5 -1 0 1 1.5 2]  OutputValues=Imax*[-10 -2 -1 0 1 2 10]
  Look-Up Table2 : Lookup  InputValues=Lc*Imax*[-2 -1.5 -1 0 1 1.5 2]  OutputValues=Imax*[-10 -2 -1 0 1 2 10]
  Sum1 : Sum  Inputs=+-  SaturateOnIntegerOverflow=on
  Sum2 : Sum  Inputs=+-  SaturateOnIntegerOverflow=on
  Sum4 : Sum  Inputs=+-  SaturateOnIntegerOverflow=on
  ia : Outport  Port=1  InitialOutput=0
  ib : Outport  Port=2  InitialOutput=0
  ic : Outport  Port=3  InitialOutput=0
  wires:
  Gain3/1 -> Sum4/2
  Sum4/1 -> Integrator/1
  Integrator/1 -> Look-Up Table/1
  a/1 -> Sum4/1
  Gain1/1 -> Sum1/2
  Sum1/1 -> Integrator1/1
  Integrator1/1 -> Look-Up Table1/1
  b/1 -> Sum1/1
  Gain5/1 -> Sum2/2
  Sum2/1 -> Integrator2/1
  Integrator2/1 -> Look-Up Table2/1
  c/1 -> Sum2/1
  Look-Up Table/1 -> Gain3/1, ia/1
  Look-Up Table1/1 -> Gain1/1, ib/1
  Look-Up Table2/1 -> Gain5/1, ic/1

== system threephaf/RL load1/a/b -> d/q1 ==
  vect : Inport  Port=1  PortDimensions=-1  SampleTime=-1  DataType=auto
  angle : Inport  Port=2  PortDimensions=-1  SampleTime=-1  DataType=auto
  Fcn_x : Fcn  Expr=u[1]*cos(u[3])-u[2]*sin(u[3])
  Fcn_y : Fcn  Expr=u[1]*sin(u[3])+u[2]*cos(u[3])
  Mux : Mux  Inputs=2
  Mux1 : Mux  Inputs=2
  Out : Outport  Port=1  InitialOutput=0
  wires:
  vect/1 -> Mux/1
  angle/1 -> Mux/2
  Mux/1 -> Fcn_x/1, Fcn_y/1
  Fcn_x/1 -> Mux1/1
  Fcn_y/1 -> Mux1/2
  Mux1/1 -> Out/1

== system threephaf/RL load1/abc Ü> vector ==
  a : Inport  Port=1  PortDimensions=-1  SampleTime=-1  DataType=auto
  b : Inport  Port=2  PortDimensions=-1  SampleTime=-1  DataType=auto
  c : Inport  Port=3  PortDimensions=-1  SampleTime=-1  DataType=auto
  Fcn : Fcn  Expr=sqrt(3/2)*u[1]
  Fcn1 : Fcn  Expr=sqrt(1/2)*(u[1]-u[2])
  Gain : Gain  Gain=1/3  Multiplication=Element-wise(K.*u)  SaturateOnIntegerOverflow=on
  Mux5 : Mux  Inputs=2
  Mux7 : Mux  Inputs=2
  Sum2 : Sum  Inputs=+++  SaturateOnIntegerOverflow=on
  Ü> ua : Sum  Inputs=+-  SaturateOnIntegerOverflow=on
  Ü> ub : Sum  Inputs=+-  SaturateOnIntegerOverflow=on
  Ü> uc : Sum  Inputs=+-  SaturateOnIntegerOverflow=on
  vect : Outport  Port=1  InitialOutput=0
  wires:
  Fcn1/1 -> Mux5/2
  Fcn/1 -> Mux5/1
  Mux5/1 -> vect/1
  Mux7/1 -> Fcn1/1
  Ü> uc/1 -> Mux7/2
  Ü> ub/1 -> Mux7/1
  Ü> ua/1 -> Fcn/1
  Gain/1 -> Ü> uc/2, Ü> ub/2, Ü> ua/2
  a/1 -> Ü> ua/1, Sum2/1
  b/1 -> Ü> ub/1, Sum2/2
  Sum2/1 -> Gain/1
  c/1 -> Ü> uc/1, Sum2/3

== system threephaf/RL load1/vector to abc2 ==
  vect : Inport  Port=1  PortDimensions=-1  SampleTime=-1  DataType=auto
  Ü> a : Fcn  Expr=sqrt(2/3)*u[1]
  Ü> b : Fcn  Expr=-sqrt(1/6)*u[1]+sqrt(1/2)*u[2]
  Ü> c : Fcn  Expr=-sqrt(1/6)*u[1]-sqrt(1/2)*u[2]
  a : Outport  Port=1  InitialOutput=0
  b : Outport  Port=2  InitialOutput=0
  c : Outport  Port=3  InitialOutput=0
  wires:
  vect/1 -> Ü> b/1, Ü> a/1, Ü> c/1
  Ü> b/1 -> b/1
  Ü> c/1 -> c/1
  Ü> a/1 -> a/1
